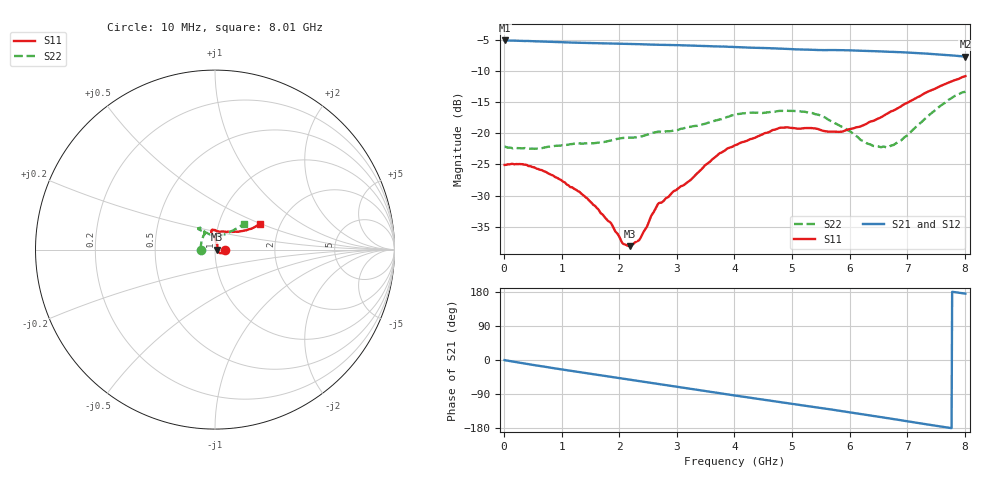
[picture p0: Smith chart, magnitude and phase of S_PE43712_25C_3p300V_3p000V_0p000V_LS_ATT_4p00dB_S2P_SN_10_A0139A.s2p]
! DEVICE ID: PE43712
! File Path: z:\PE43713\PE43713_CHAR_NOM_04292014\AMB\3p300\LS_ATT_4p00dB\PE43713_AMB_3p300V_3p000V_0p000V_LS_ATT_4p00dB_S2P_SN_10_A0139A.s2p
! Serial: 10
! Lot: A0139A
! Temp: 25C
! VDD: 3.300
! VSS: 0.000
! Control_Hi: 3.000
! Control_Lo: 0.000
! Attenuation Step: 4.00dB
! Port 1: RF1
! Port 2: RF2
! ThroughPath:1-2
! IDD: 0.0001468859
! ISS: -4.23e-008
#  Hz  S  RI  R  50
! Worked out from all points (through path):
!   801 points, 10 MHz to 8.01 GHz, reference 50 ohm
!   highest |S21| = -5.09 dB at 10 MHz (marker M1); lowest = -7.7 dB at 8.01 GHz (marker M2)
!   group delay of S21, straight-line fit = 63.4 ps
!   lowest |S11| = -38.1 dB at 2.18 GHz (marker M3), VSWR 1.03, Z = 51.3 + j0.0122 ohm
!   |S11| at or under -10 dB: start of sweep to end of sweep
!   |S22| runs from -22.5 to -13.3 dB; largest |S21 - S12| = 0.0017
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1e7  0.0557 -0.000149  0.5565 -0.00323  0.5562 -0.00298  -0.0781 0.000401
3.4e8  0.055 -0.0115  0.5446 -0.085  0.5442 -0.0837  -0.0756 0.00449
6.3e8  0.0478 -0.0174  0.525 -0.1506  0.5249 -0.1507  -0.0752 0.00944
9.6e8  0.0377 -0.0202  0.4932 -0.2187  0.4933 -0.2187  -0.078 0.0163
1.35e9  0.0264 -0.0189  0.4473 -0.289  0.4473 -0.289  -0.0788 0.0256
1.85e9  0.0171 -0.00872  0.3764 -0.3668  0.3764 -0.3667  -0.0758 0.0435
2.07e9  0.0126 -0.0032  0.3409 -0.3965  0.341 -0.3964  -0.0761 0.0512
2.18e9  0.0124 0.000119  0.3224 -0.4101  0.3225 -0.4098  -0.0743 0.055
2.36e9  0.0119 0.00779  0.2902 -0.4304  0.2902 -0.4302  -0.0692 0.0633
2.68e9  0.0143 0.0232  0.2317 -0.4586  0.2317 -0.4587  -0.06 0.0841
3.22e9  0.0055 0.0412  0.1251 -0.4911  0.1252 -0.4912  -0.0602 0.0951
3.72e9  -0.000533 0.0677  0.0259 -0.4974  0.0257 -0.4973  -0.0651 0.1107
4.01e9  -0.00831 0.0796  -0.0317 -0.4922  -0.0316 -0.4922  -0.0764 0.1187
4.79e9  -0.0185 0.1093  -0.1727 -0.4461  -0.1727 -0.4464  -0.0926 0.1197
5.35e9  -0.00484 0.1098  -0.2578 -0.391  -0.2577 -0.3908  -0.0915 0.113
5.63e9  0.0101 0.1026  -0.2957 -0.36  -0.2956 -0.3602  -0.075 0.1046
5.86e9  0.0251 0.0999  -0.3276 -0.3301  -0.3272 -0.3301  -0.0577 0.0973
6.32e9  0.0696 0.0996  -0.3774 -0.2602  -0.3765 -0.26  -0.0178 0.0804
6.68e9  0.1078 0.099  -0.4056 -0.1982  -0.4052 -0.1981  0.0162 0.076
6.9e9  0.1323 0.0997  -0.4186 -0.1588  -0.4182 -0.1588  0.0383 0.0796
7.71e9  0.2212 0.1258  -0.4239 -0.0113  -0.4236 -0.0117  0.1348 0.1265
8.01e9  0.2504 0.1417  -0.4116 0.0353  -0.4109 0.0345  0.1614 0.1438
